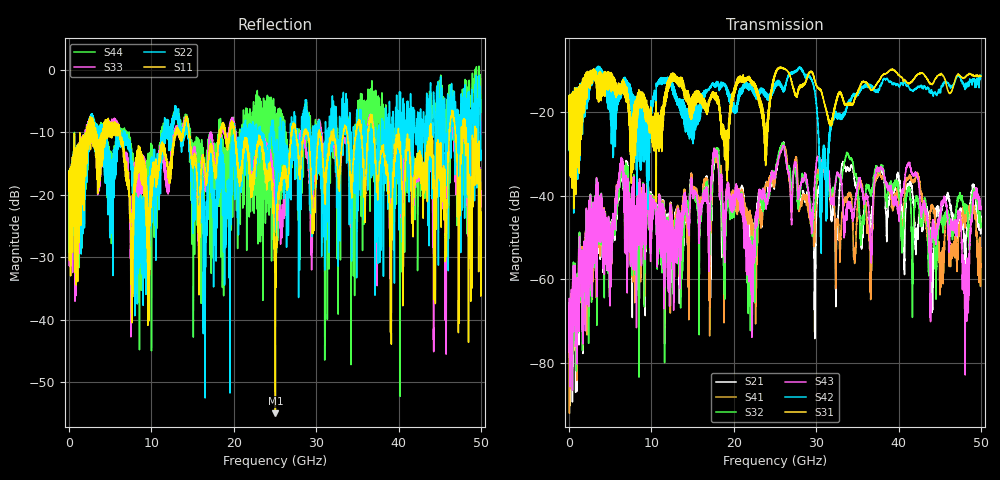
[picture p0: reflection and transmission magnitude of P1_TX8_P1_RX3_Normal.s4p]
!Keysight Technologies,N5225B,MY57041031,A.13.20.10
!Date: Friday, May 31, 2019 11:17:52
!Correction: S11(Full 4 Port(1,2,3,4))
!S12(Full 4 Port(1,2,3,4))
!S13(Full 4 Port(1,2,3,4))
!S14(Full 4 Port(1,2,3,4))
!S21(Full 4 Port(1,2,3,4))
!S22(Full 4 Port(1,2,3,4))
!S23(Full 4 Port(1,2,3,4))
!S24(Full 4 Port(1,2,3,4))
!S31(Full 4 Port(1,2,3,4))
!S32(Full 4 Port(1,2,3,4))
!S33(Full 4 Port(1,2,3,4))
!S34(Full 4 Port(1,2,3,4))
!S41(Full 4 Port(1,2,3,4))
!S42(Full 4 Port(1,2,3,4))
!S43(Full 4 Port(1,2,3,4))
!S44(Full 4 Port(1,2,3,4))
!S4P File: Measurements: <S11,S12,S13,S14>,
!<S21,S22,S23,S24>,
!<S31,S32,S33,S34>,
!<S41,S42,S43,S44>:
# Hz S  dB  R 50.0
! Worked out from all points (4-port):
!   5000 points, 10 MHz to 50 GHz, reference 50 ohm
!   strongest paths, dB at 10 MHz, 12.51 GHz, 25.01 GHz, 37.51 GHz, 50 GHz:
!     S31: -19.7, -10.8, -11.0, -12.6, -11.3
!     S42: -19.5, -14.4, -13.3, -15.0, -11.1
!     S43: -66.5, -47.4, -35.1, -34.2, -42.6
!     S32: -65.7, -48.2, -34.4, -33.9, -47.1
!     S41: -71.6, -47.2, -35.9, -35.0, -52.5
!     S21: -72.8, -47.0, -36.2, -35.3, -46.9
!   lowest |S11| = -55.0 dB at 25.05 GHz (marker M1), VSWR 1.00, Z = 49.8 + j0.00744 ohm
!   |S11| at or under -10 dB: 6.192 GHz to 12.89 GHz (6.695 GHz wide, 70.2 % of centre); 20.1 GHz to 26.99 GHz (6.892 GHz wide, 29.3 % of centre); 40 GHz to 43.77 GHz (3.765 GHz wide, 8.99 % of centre)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
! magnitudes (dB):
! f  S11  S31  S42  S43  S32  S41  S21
! 10 MHz  -19.4  -19.7  -19.5  -66.5  -65.7  -71.6  -72.8
! 6.35 GHz  -11.8  -14.4  -15.0  -30.8  -32.2  -31.3  -32.7
! 17.97 GHz  -13.4  -16.2  -12.6  -29.6  -28.5  -31.3  -30.2
! 21.89 GHz  -16.2  -11.5  -13.3  -56.8  -58.1  -45.5  -48.6
! 25.05 GHz  -55.0  -10.5  -13.5  -34.1  -34.1  -34.7  -35.4
! 30.63 GHz  -11.2  -14.9  -40.8  -32.1  -33.3  -32.6  -35.7
! 50 GHz  -22.8  -11.3  -11.1  -42.6  -47.1  -52.5  -46.9
